TEXTLIST SystemDisplay
  1 = 'Window XP' | chinese: 'Window XP' | english: 'Window XP'
  2 = 'U盘' | chinese: 'U盘' | english: 'USB Device'
  3 = 'Window CE' | chinese: 'Window CE' | english: 'Window CE'
   = ''
END_TEXTLIST
